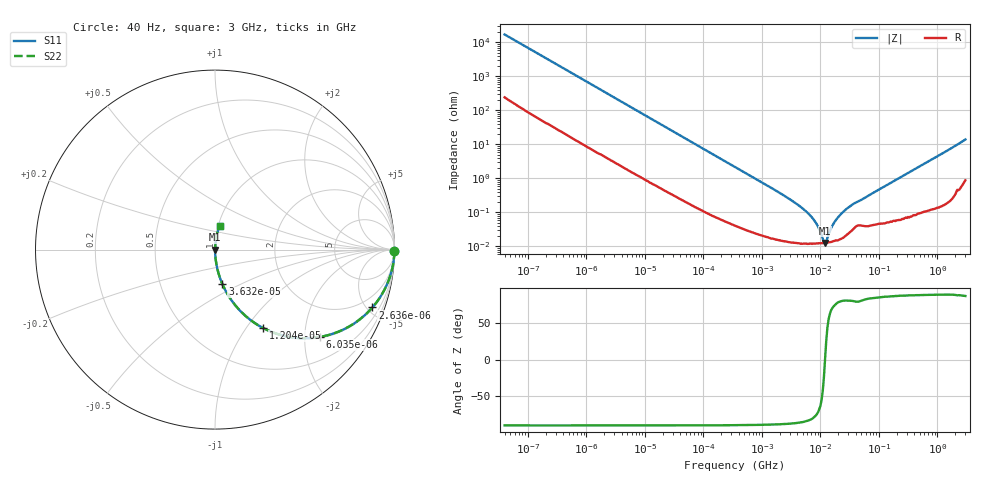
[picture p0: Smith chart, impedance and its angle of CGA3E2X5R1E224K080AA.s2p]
! S-parameter Generated by TDK Corporation
! Copyright(C) 2015 TDK Corporation.
! All Rights Reserved.
! TDK P/N: CGA3E2X5R1E224K080AA (Multilayer Ceramic Chip Capacitors)
! Property: C=220nF
! Size(LxWxT): 1.6x0.8x0.8mm, 0.063x0.031x0.031inches
! Model Type: s2p (Touchstone File Format Version 1.0)
! Frequency: DC=Yes Start=0.00004MHz Stop=3000MHz 396points Log-sweep
! Note: This model was converted from impedance.
! Model Generated on Jun. 23, 2015
! Hash(MD5):
! Port Assignments:
!  1 ---| |--- 2
! Applicable Conditions:
!  Temperature = 25 degC
!  DC Bias Voltage = 0 V
!  Small Signal Operation
! Terms and conditions regarding TDK Simulation Models
! (1)This simulation model is being provided solely for informational purposes. Please refer to the specifications of the products in terms of detailed characteristics of such products.
! (2)In no event shall TDK Corporation of any of its subsidiaries be liable for any loss or damage arising, directly or indirectly,
!  From any information contained in this simulation model, including, but not limited to loss or damages arising from any inaccuracies, omissions or errors in connection with such information.
! (3)Any and all copyrights on this simulation model are owned by TDK Corporation.
!  Duplication or redistribution of this simulation model without prior written permission from TDK Corporation is prohibited.
! (4)This simulation model is subject to any modification or change without any prior notice.
! (5)Neither TDK Corporation nor any of its subsidiaries shall make any warranty, express or implied,
!  Including but not limited to the correctness, implied warranties of merchantability and fitness for a particular purpose with respect to this simulation models.
! (6)The use of this simulation model shall be deemed to have consented to the terms and conditions hereof.
# MHz S MA R 50
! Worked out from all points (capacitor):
!   395 points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, 40 Hz to 3 GHz, reference 50 ohm
!   read as one part in series: C = 231 nF near 41.88 Hz
!   lowest |Z| = 12.5 mohm at 11.98 MHz (marker M1)
!   series resonance near 11.96 MHz, so ESL is about 770 pH
!   S11 on the Smith chart (normalised r, x): 40 Hz: open; 2.636 kHz: 1.07, -5.42; 6.035 kHz: 1.03, -2.38; 12.04 kHz: 1.02, -1.20; 36.32 kHz: 1.01, -0.40; 3 GHz: 1.02, +0.28
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4e-05  0.9999 -0.3  0.005822 88.9  0.005822 88.9  0.9999 -0.3
0.0002520917  0.9989 -2.1  0.03585 87.2  0.03585 87.2  0.9989 -2.1
0.000834128  0.9917 -6.7  0.1167 82.6  0.1167 82.6  0.9917 -6.7
0.002635842  0.9344 -20.2  0.3449 69.1  0.3449 69.1  0.9344 -20.2
0.006035228  0.7612 -39.7  0.6392 49.6  0.6392 49.6  0.7612 -39.7
0.01203665  0.5119 -58.5  0.8527 30.8  0.8527 30.8  0.5119 -58.5
0.01739424  0.383 -66.7  0.9188 22.5  0.9188 22.5  0.383 -66.7
0.03632493  0.1969 -77.9  0.9778 11.4  0.9778 11.4  0.1969 -77.9
0.09548642  0.07749 -84.7  0.9959 4.4  0.9959 4.4  0.07749 -84.7
0.3464102  0.02179 -87.7  0.9994 1.2  0.9994 1.2  0.02179 -87.7
2.877491  0.00253 -86.9  0.9999 0.1  0.9999 0.1  0.00253 -86.9
4.998775  0.001283 -84.6  0.9999 0.1  0.9999 0.1  0.001283 -84.6
7.22376  0.0006914 -80.2  0.9999 0.0  0.9999 0.0  0.0006914 -80.2
9.092863  0.0003796 -71.3  0.9999 0.0  0.9999 0.0  0.0003796 -71.3
11.44558  0.0001368 -24.4  0.9999 0.0  0.9999 0.0  0.0001368 -24.4
11.98465  0.0001255 1.0  0.9999 -0.0  0.9999 -0.0  0.0001255 1.0
16.54008  0.0004483 71.6  0.9999 -0.0  0.9999 -0.0  0.0004483 71.6
25.02793  0.001069 80.1  0.9998 -0.1  0.9998 -0.1  0.001069 80.1
37.87146  0.001831 79.2  0.9997 -0.1  0.9997 -0.1  0.001831 79.2
150.6385  0.006971 85.4  0.9995 -0.4  0.9995 -0.4  0.006971 85.4
994.0817  0.04416 85.7  0.9977 -2.5  0.9977 -2.5  0.04416 85.7
3000  0.1369 78.6  0.982 -7.9  0.982 -7.9  0.1369 78.6
